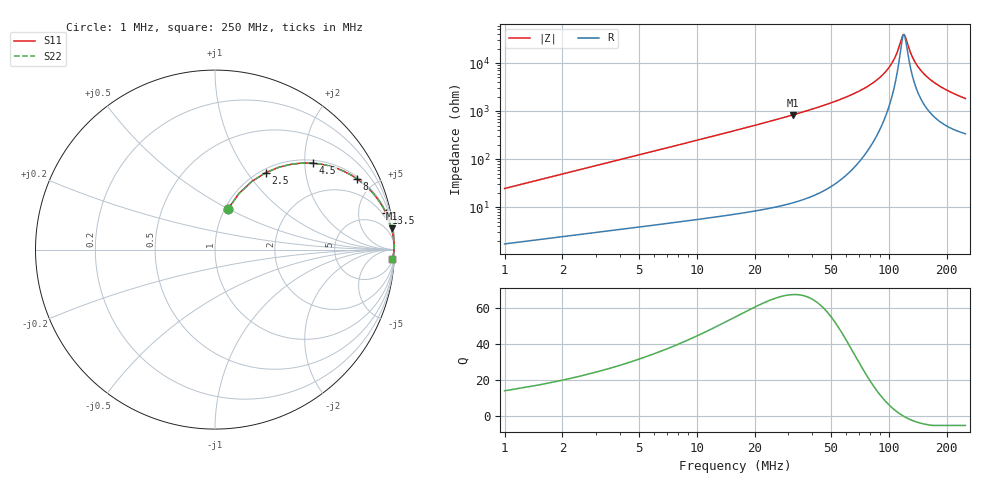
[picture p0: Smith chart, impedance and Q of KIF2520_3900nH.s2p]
!version-2
!date-12.2020
!Series
# MHz S RI R 50
!Freq ReS11 ImS11 ReS21 ImS21 ReS12 ImS12 ReS22 ImS22
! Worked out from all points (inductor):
!   499 points, 1 MHz to 250 MHz, reference 50 ohm
!   read as one part in series: L = 3.9 uH near 2 MHz
!   highest Q = 67.4 at 31.5 MHz (marker M1), where L = 4.19 uH
!   self-resonance near 119.5 MHz
!   S11 on the Smith chart (normalised r, x): 1 MHz: 1.03, +0.49; 2.5 MHz: 1.05, +1.23; 4.5 MHz: 1.07, +2.21; 8 MHz: 1.10, +3.94; 18.5 MHz: 1.16, +9.29; 250 MHz: 8, -36
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1  0.0709 0.2238  0.9291 -0.2238  0.9291 -0.2238  0.0709 0.2238
2.5  0.2821 0.4283  0.7179 -0.4283  0.7179 -0.4283  0.2821 0.4283
4.5  0.5481 0.4813  0.4519 -0.4813  0.4519 -0.4813  0.5481 0.4813
6  0.6802 0.4522  0.3198 -0.4522  0.3198 -0.4522  0.6802 0.4522
8  0.7892 0.3955  0.2108 -0.3955  0.2108 -0.3955  0.7892 0.3955
12  0.8933 0.2985  0.1067 -0.2985  0.1067 -0.2985  0.8933 0.2985
18.5  0.9525 0.2043  0.0475 -0.2043  0.0475 -0.2043  0.9525 0.2043
31.5  0.984 0.1184  0.016 -0.1184  0.016 -0.1184  0.984 0.1184
42.5  0.9917 0.0831  0.00829 -0.0831  0.00829 -0.0831  0.9917 0.0831
84  0.9979 0.0245  0.00212 -0.0245  0.00212 -0.0245  0.9979 0.0245
95.5  0.998 0.0154  0.00203 -0.0154  0.00203 -0.0154  0.998 0.0154
104  0.9979 0.00957  0.00212 -0.00957  0.00212 -0.00957  0.9979 0.00957
110  0.9978 0.00575  0.00225 -0.00575  0.00225 -0.00575  0.9978 0.00575
118.5  0.9975 0.00071  0.0025 -0.00071  0.0025 -0.00071  0.9975 0.00071
121  0.9974 -0.000699  0.00259 0.000699  0.00259 0.000699  0.9974 -0.000699
125.5  0.9972 -0.00316  0.00277 0.00316  0.00277 0.00316  0.9972 -0.00316
132.5  0.9969 -0.00682  0.00308 0.00682  0.00308 0.00682  0.9969 -0.00682
141  0.9965 -0.011  0.00351 0.011  0.00351 0.011  0.9965 -0.011
152.5  0.9958 -0.0164  0.00418 0.0164  0.00418 0.0164  0.9958 -0.0164
167  0.9949 -0.0227  0.00514 0.0227  0.00514 0.0227  0.9949 -0.0227
208.5  0.9914 -0.0386  0.00855 0.0386  0.00855 0.0386  0.9914 -0.0386
250  0.9872 -0.0525  0.0128 0.0525  0.0128 0.0525  0.9872 -0.0525
